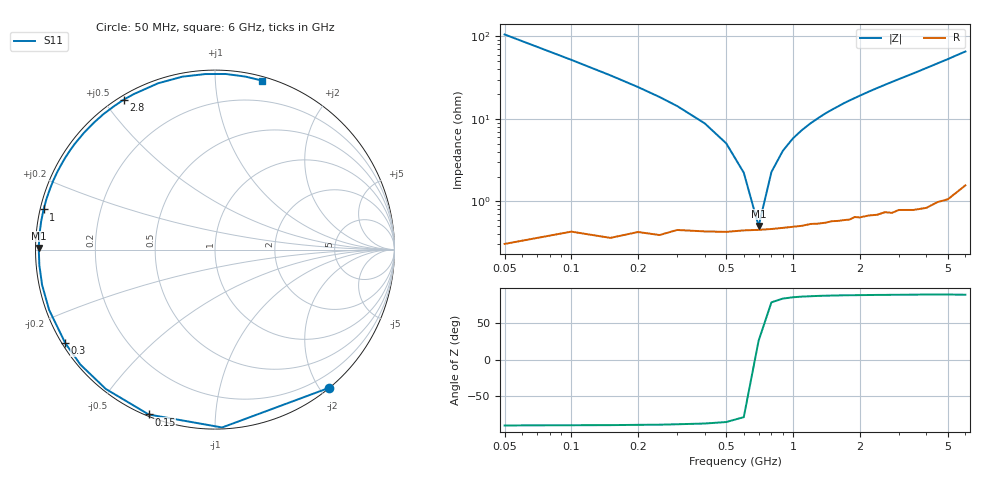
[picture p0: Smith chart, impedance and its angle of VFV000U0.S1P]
! Infineon Technologies  Discrete & RF Semiconductors
! BBY 58-03
! Si Tuning Diode in SOD323
! VR = 0 V
! S-Parameters:  June  1999
# GHz  S  MA  R  50
!  f  S11
! GHz  MAG  ANG
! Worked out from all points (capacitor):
!   34 points, 50 MHz to 6 GHz, reference 50 ohm
!   read as one part to ground: C = 29.9 pF near 50 MHz
!   lowest |Z| = 501 mohm at 700 MHz (marker M1)
!   series resonance near 690.9 MHz, so ESL is about 1.8 nH
!   S11 on the Smith chart (normalised r, x): 50 MHz: 0.01, -2.12; 150 MHz: 0.01, -0.68; 300 MHz: 0.01, -0.29; 1 GHz: 0.01, +0.12; 2.8 GHz: 0.01, +0.56; 6 GHz: 0.03, +1.31
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0.05  0.9978 -50.6
0.1  0.9918 -87.7
0.15  0.9902 -111.9
0.2  0.9864 -128.1
0.25  0.9864 -139.5
0.3  0.9835 -148.0
0.4  0.9834 -160.0
0.5  0.9833 -168.5
0.6  0.9824 -175.0
0.7  0.9821 179.5
0.8  0.9817 174.9
1  0.9808 166.8
1.1  0.9804 163.3
1.3  0.9796 156.9
1.4  0.9793 153.8
1.6  0.9788 148.3
1.8  0.9786 143.0
2  0.978 138.2
2.2  0.9775 133.6
2.4  0.9778 129.3
2.8  0.9782 121.3
3  0.9773 117.5
3.5  0.9794 108.9
4  0.9804 100.7
4.5  0.9795 93.2
5  0.9803 86.5
5.5  0.9788 80.1
6  0.9774 74.5
